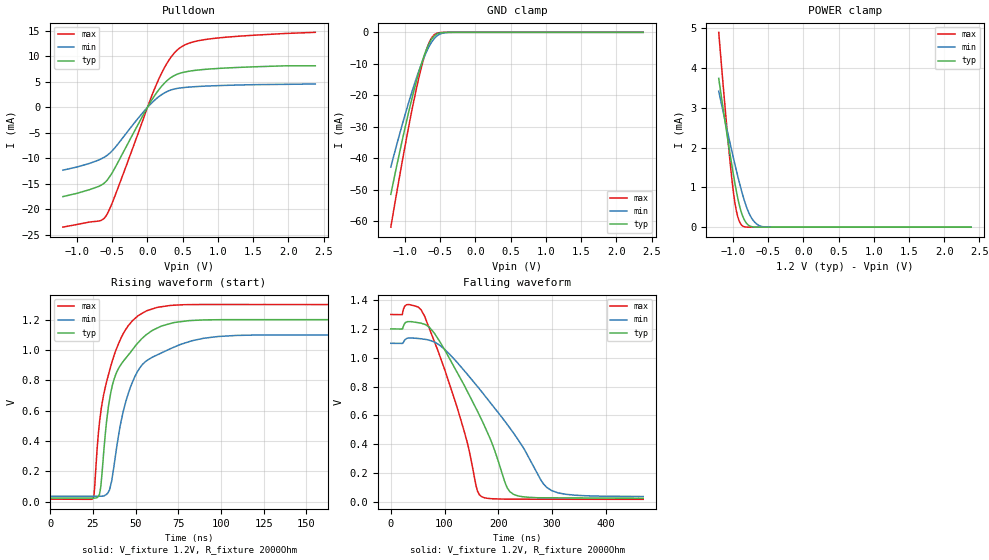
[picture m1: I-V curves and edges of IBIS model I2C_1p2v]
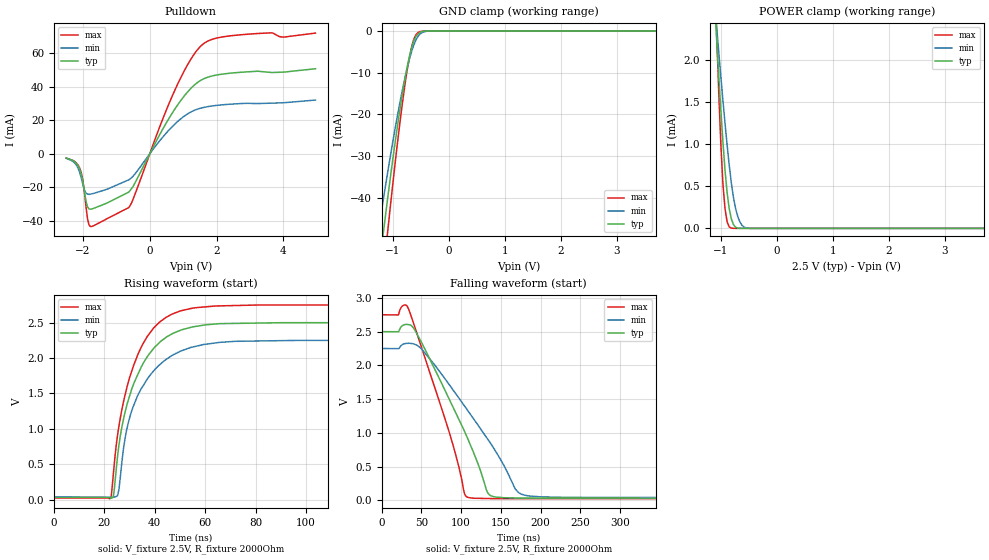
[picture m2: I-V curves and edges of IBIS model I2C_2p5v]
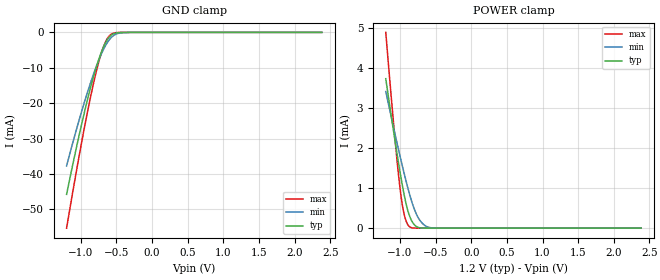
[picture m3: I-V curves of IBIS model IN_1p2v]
|Texas Instruments Incorporated
|Ultra Low Power Stereo Audio Codec with miniDSP, DirectPath Headphone,
| and Stereo Class-D Speaker Amplifier
|part#   Digital Voltage Range   Package-type   #pin
|TLV320AIC3212   1.1V to 3.6V   WCSP   81
[IBIS Ver]   4.0
[File name]   tlv320aic3212.ibs
[File Rev]   1.0
[Date]   09/07/2011
[Source]   Texas Instruments Incorporated.
   Analog-eLab, HPA
   12500 TI Blvd
   Dallas, TX -75243
   For Support e-mail: elab_ibis@list.ti.com
[Notes]   Revision History:
   1.0: 09/07/2011
- Initial version of the model
- Initial Model generated from simulations.
- Model not matched to measurements
- ccomp values are based on PVT conditions although listed in numerical order.
- Model names with a trailing _1p2v contains the model for 1.2V operaton.
- Model names with a trailing _1p8v contains the model for 1.8V operaton.
- Model names with a trailing _2p5v contains the model for 2.5V operaton.
- Model names with a trailing _3p3v contains the model for 3.3V operaton.
- Non monotinicity warnings related to combined Pullup/Pulldown of INOUT_xxxx and I2C_xxxx
  reflect the simulationresults.
[Disclaimer]
 This product is designed as an aid for customers of Texas Instruments.
 No warranties, either expressed or implied, with respect to this third
 party software (if any) or with respect to its fitness for any
 particular purpose is claimed by Texas Instruments or the author. The
 software (if any) is provided solely on an "as is" basis. The entire
 risk as to its quality and performance is with the customer
[Copyright] (C) Copyright 2012 Texas Instruments Incorporated.
   All rights reserved.
|   TLV320AIC3212
[Component]   tlv320aic3212
[Manufacturer] TI
[Package]   | 81 pin  package
| variable   typ   min   max
R_pkg   0.01   0.008   0.012
L_pkg   0.1nH   0.08nH   0.12nH
C_pkg   0.1pF   0.08pF   0.12pF
|-------------------------PIN------------------------------------------------
[Pin]   signal_name  model_name  R_pin  L_pin C_pin
A1   AVDD3_33   POWER   NA   NA   NA
A2   RECVSS   GND   NA   NA   NA
A3   RECVDD_33   POWER   NA   NA   NA
A4   HPR   TERM   NA   NA   NA
A5   VNEG   TERM   NA   NA   NA
A6   CPFCM   TERM   NA   NA   NA
A7   CPVDD_18   POWER   NA   NA   NA
A8   AVSS4   GND   NA   NA   NA
A9   SPKLP   TERM   NA   NA   NA
B1   MICDET   TERM   NA   NA   NA
B2   RECP   TERM   NA   NA   NA
B3   RECM   TERM   NA   NA   NA
B4   HVDD_18   POWER   NA   NA   NA
B5   HPL   TERM   NA   NA   NA
B6   CPVSS   GND   NA   NA   NA
B7   CPFCP   TERM   NA   NA   NA
B8   SLVDD   POWER   NA   NA   NA
B9   SLVSS   GND   NA   NA   NA
C1   IN4L   TERM   NA   NA   NA
C2   AVDD1_18   POWER   NA   NA   NA
C3   MICBIAS_EXT   TERM   NA   NA   NA
C4   MICBIAS   TERM   NA   NA   NA
C5   AVDD2_18   POWER   NA   NA   NA
C6   LOL   TERM   NA   NA   NA
C7   AVDD4_18   POWER   NA   NA   NA
C8   SPKLM   TERM   NA   NA   NA
C9   SPKRM   TERM   NA   NA   NA
D1   VREF_AUDIO   TERM   NA   NA   NA
D2   VREF_SAR   TERM   NA   NA   NA
D3   IN1L_AUX1   TERM   NA   NA   NA
D4   IN1R_AUX2   TERM   NA   NA   NA
D5   IN4R   TERM   NA   NA   NA
D6   HPVSS_SENSE   TERM   NA   NA   NA
D7   LOR   TERM   NA   NA   NA
D8   SRVSS   GND   NA   NA   NA
D9   SRVDD   POWER   NA   NA   NA
E1   IN3R   TERM   NA   NA   NA
E2   IN3L   TERM   NA   NA   NA
E3   AVSS   GND   NA   NA   NA
E4   AVSS1   GND   NA   NA   NA
E5   AVSS3   GND   NA   NA   NA
E6   AVSS2   GND   NA   NA   NA
E7   DVSS   GND   NA   NA   NA
E8   SPK_V   POWER   NA   NA   NA
E9   SPKRP   TERM   NA   NA   NA
F1   IN2L   TERM   NA   NA   NA
F2   IN2R   TERM   NA   NA   NA
F3   AVDD_18   POWER   NA   NA   NA
F4   DVSS   GND   NA   NA   NA
F5   GPI3   IN_PD   NA   NA   NA
F6   GPI2   IN   NA   NA   NA
F7   GPI4   IN_PD   NA   NA   NA
F8   IOVSS   GND   NA   NA   NA
F9   VBAT   TERM   NA   NA   NA
G1   MCLK1   IN   NA   NA   NA
G2   BCLK2   INOUT   NA   NA   NA
G3   DIN2   IN   NA   NA   NA
G4   WCLK2   INOUT   NA   NA   NA
G5   WCLK3   INOUT   NA   NA   NA
G6   DIN3   IN   NA   NA   NA
G7   SPI_SELECT  IN_PD   NA   NA   NA
G8   RESETB   IN   NA   NA   NA
G9   MCLK2   IN   NA   NA   NA
H1   BCLK1   INOUT   NA   NA   NA
H2   DOUT1   OUT_HOLD   NA   NA   NA
H3   IOVDD   POWER   NA   NA   NA
H4   SCL   I2C_IO   NA   NA   NA
H5   SDA   I2C_IO   NA   NA   NA
H6   GPO1   OUT   NA   NA   NA
H7   BCLK3   INOUT   NA   NA   NA
H8   GPIO2   INOUT   NA   NA   NA
H9   IOVDD   POWER   NA   NA   NA
J1   DIN1   IN   NA   NA   NA
J2   WCLK1   INOUT   NA   NA   NA
J3   DVDD   POWER   NA   NA   NA
J4   IOVSS   GND   NA   NA   NA
J5   GPI1   IN   NA   NA   NA
J6   DOUT2   OUT_HOLD   NA   NA   NA
J7   DOUT3   OUT_HOLD   NA   NA   NA
J8   GPIO1   INOUT   NA   NA   NA
J9   DVDD   POWER   NA   NA   NA
[Model Selector] I2C_IO
I2C_3p3v   I2C I/O with 3.3V operation.
I2C_2p5v   I2C I/O with 2.5V operation.
I2C_1p8v   I2C I/O with 1.8V operation.
I2C_1p2v   I2C I/O with 1.2V operation.
[Model Selector] IN
IN_3p3v   Input with 3.3V operation.
IN_2p5v   Input with 2.5V operation.
IN_1p8v   Input with 1.8V operation.
IN_1p2v   Input with 1.2V operation.
[Model Selector] IN_PD
IN_PD_3p3v  Input with 3.3V operation.
IN_PD_2p5v  Input with 2.5V operation.
IN_PD_1p8v  Input with 1.8V operation.
IN_PD_1p2v  Input with 1.2V operation.
[Model Selector] INOUT
INOUT_3p3v   I/O with 3.3V operation.
INOUT_2p5v   I/O with 2.5V operation.
INOUT_1p8v   I/O with 1.8V operation.
INOUT_1p2v   I/O with 1.2V operation.
[Model Selector] OUT
OUT_3p3v   Output with 3.3V operation.
OUT_2p5v   Output with 2.5V operation.
OUT_1p8v   Output with 1.8V operation.
OUT_1p2v   Output with 1.2V operation.
[Model Selector] OUT_HOLD
OUT_HOLD_3p3v   Output with 3.3V operation.
OUT_HOLD_2p5v   Output with 2.5V operation.
OUT_HOLD_1p8v   Output with 1.8V operation.
OUT_HOLD_1p2v   Output with 1.2V operation.
[Model Selector] TERM
TERM_3p3v   Termination with 3.3V operation.
TERM_2p5v   Termination with 2.5V operation.
TERM_1p8v   Termination with 1.8V operation.
TERM_1p2v   Termination with 1.2V operation.
|   TERM_1p2v
[Model]  TERM_1p2v
Model_type Terminator
C_comp   1fF   1fF   1fF
[Voltage Range]  1.2   1.1  1.3
[Temperature Range] 27   125   -40
|   TERM_1p8v
[Model]  TERM_1p8v
Model_type Terminator
C_comp   1fF   1fF   1fF
[Voltage Range]  1.8   1.65  1.95
[Temperature Range] 27   125   -40
|   TERM_2p5v
[Model]  TERM_2p5v
Model_type Terminator
C_comp   1fF   1fF   1fF
[Voltage Range]  2.5   2.25  2.75
[Temperature Range] 27   125   -40
|   TERM_3p3v
[Model]  TERM_3p3v
Model_type Terminator
C_comp   1fF   1fF   1fF
[Voltage Range]  3.3   2.7  3.6
[Temperature Range] 27   125   -40
| Models and submodels in the file (28): I2C_1p2v (I/O_open_drain), I2C_1p8v (I/O_open_drain), I2C_2p5v (I/O_open_drain), I2C_3p3v (I/O_open_drain), IN_1p2v (Input), IN_1p8v (Input), IN_2p5v (Input), IN_3p3v (Input), IN_PD_1p2v (Input), IN_PD_1p8v (Input), IN_PD_2p5v (Input), IN_PD_3p3v (Input), INOUT_1p2v (I/O), INOUT_1p8v (I/O), INOUT_2p5v (I/O), INOUT_3p3v (I/O), OUT_1p2v (Output), OUT_1p8v (Output), OUT_2p5v (Output), OUT_3p3v (Output), OUT_HOLD_1p2v (Output), OUT_HOLD_1p8v (Output), OUT_HOLD_2p5v (Output), OUT_HOLD_3p3v (Output), TERM_1p2v (Terminator), TERM_1p8v (Terminator), TERM_2p5v (Terminator), TERM_3p3v (Terminator)
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|   I2C_1p2v
[Model]   I2C_1p2v
Model_type   I/O_open_drain
Polarity   Non-Inverting
Enable   Active-High
Vinl = 0.12
Vinh = 1.08
Vmeas = 0.6
Vref = 0
Cref = 5pF
Rref = 2000
|   typ   min   max
C_comp   1.274pF   1.219pF   1.333pF
[Voltage Range]   1.2   1.1   1.3
[Temperature Range]   27   125   -40
[Pullup Reference]   1.2   1.1   1.3
[Pulldown Reference]   -0   -0   -0
[Power Clamp Reference]   1.2   1.1   1.3
[GND Clamp Reference]   -0   -0   -0
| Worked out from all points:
|   slope of the pulldown table from 0 to 0.18 V, typ, clamps not added: 47.5 ohm
|   GND clamp passes 1 mA (typ) near -0.58 V on its own axis
|   POWER clamp passes 1 mA (typ) near -0.96 V on its own axis
|   falling waveform, V_fixture 1.2V, R_fixture 2000Ohm: 20-80 % time 88.3ns typ, 123ns min, 62.1ns max; typ from 1.2 V to 0.024 V
|   rising waveform, V_fixture 1.2V, R_fixture 2000Ohm: 20-80 % time 14.7ns typ, 15.2ns min, 13.1ns max; typ from 0.024 V to 1.2 V
[Pulldown]
|   Voltage   I(typ)   I(min)   I(max)
-1.2V     -17.52mA   -12.33mA   -23.52mA
-660mV    -15.3mA    -10.14mA   -22.22mA
-588mV    -14.55mA   -9.571mA   -21.32mA
-534mV    -13.56mA   -8.98mA    -19.87mA
-444mV    -11.44mA   -7.63mA    -16.76mA
-84mV     -2.1mA     -1.335mA   -3.236mA
132mV     2.914mA    1.776mA    4.67mA
294mV     5.441mA    3.206mA    9.049mA
456mV     6.677mA    3.793mA    11.64mA
636mV     7.195mA    4.032mA    12.81mA
924mV     7.575mA    4.234mA    13.51mA
2.382V    8.16mA     4.595mA    14.74mA
[GND Clamp]
|   Voltage   I(typ)   I(min)   I(max)
-1.2V     -51.53mA   -42.82mA   -61.95mA
-1.11V    -41.81mA   -35.22mA   -50.18mA
-966mV    -27.21mA   -23.77mA   -32.33mA
-894mV    -20.51mA   -18.48mA   -24.05mA
-822mV    -14.35mA   -13.57mA   -16.43mA
-750mV    -8.941mA   -9.16mA    -9.735mA
-696mV    -5.556mA   -6.287mA   -5.617mA
-642mV    -2.944mA   -3.902mA   -2.598mA
-588mV    -1.249mA   -2.113mA   -881.8uA
-498mV    -172.7uA   -521.4uA   -72.82uA
-372mV    -4.652uA   -38.41uA   -629.2nA
2.382V    0A         0A         0A
[POWER Clamp]
|   Voltage   I(typ)   I(min)   I(max)
-1.2V     3.742mA    3.419mA    4.901mA
-1.074V   2.231mA    2.387mA    2.298mA
-1.002V   1.428mA    1.82mA     1.03mA
-966mV    1.06mA     1.547mA    562.3uA
-930mV    731.2uA    1.283mA    261.4uA
-894mV    461.7uA    1.032mA    95.6uA
-858mV    267uA      798.5uA    24.83uA
-804mV    94.07uA    498uA      2.256uA
-732mV    11.82uA    224.2uA    69.47nA
-660mV    942.6nA    77.54uA    0A
-570mV    25.2nA     10.87uA    0A
2.382V    0A         0A         0A
[Ramp]
R_load = 2000
|   typ   min   max
dV/dt_r   0.705406/1.46932e-008  0.638454/1.52438e-008  0.769932/1.30398e-008
dV/dt_f   0.705409/8.81291e-008   0.63829/1.23398e-007  0.769933/6.21317e-008
[Falling Waveform]
V_fixture = 1.2V
V_fixture_min = 1.1V
V_fixture_max = 1.3V
R_fixture = 2000Ohm
C_fixture = 0F
|   Time   V(typ)   V(min)   V(max)
0s        1.2V       1.1V       1.3V
32.69ns   1.251V     1.136V     1.369V
62.72ns   1.232V     1.128V     1.29V
120.1ns   920.9mV    981.3mV    694.6mV
161.3ns   629.2mV    800.4mV    74.84mV
169.6ns   565.2mV    761.9mV    34.22mV
216.7ns   96.76mV    537mV      17.74mV
228.5ns   51.31mV    476.9mV    17.7mV
299.2ns   27.33mV    77.85mV    17.43mV
470ns     24.32mV    36.18mV    16.78mV
[Rising Waveform]
V_fixture = 1.2V
V_fixture_min = 1.1V
V_fixture_max = 1.3V
R_fixture = 2000Ohm
C_fixture = 0F
|   Time   V(typ)   V(min)   V(max)
0s        24.32mV    35.9mV     16.78mV
24.99ns   24.02mV    35.98mV    20.42mV
29.9ns    136.2mV    36mV       617.3mV
34.13ns   633.5mV    65.85mV    839.6mV
37.53ns   812.9mV    252.1mV    970.6mV
42.58ns   923.8mV    589mV      1.105V
48.06ns   1.001V     786.7mV    1.193V
62.72ns   1.146V     968.9mV    1.282V
109.1ns   1.201V     1.097V     1.301V
470ns     1.2V       1.1V       1.3V
|   I2C_2p5v
[Model]   I2C_2p5v
Model_type   I/O_open_drain
Polarity   Non-Inverting
Enable   Active-High
Vinl = 0.75
Vinh = 1.75
Vmeas = 1.25
Vref = 0
Cref = 5pF
Rref = 2000
|   typ   min   max
C_comp   1.274pF   1.219pF   1.333pF
[Voltage Range]   2.5   2.25   2.75
[Temperature Range]   27   125   -40
[Pullup Reference]   2.5   2.25   2.75
[Pulldown Reference]   -0   -0   -0
[Power Clamp Reference]   2.5   2.25   2.75
[GND Clamp Reference]   -0   -0   -0
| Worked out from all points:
|   slope of the pulldown table from 0 to 0.375 V, typ, clamps not added: 26.4 ohm
|   GND clamp passes 1 mA (typ) near -0.57 V on its own axis
|   POWER clamp passes 1 mA (typ) near -0.96 V on its own axis
|   falling waveform, V_fixture 2.5V, R_fixture 2000Ohm: 20-80 % time 57.5ns typ, 76.1ns min, 43.6ns max; typ from 2.5 V to 0.031 V
|   rising waveform, V_fixture 2.5V, R_fixture 2000Ohm: 20-80 % time 11.8ns typ, 12.5ns min, 11.3ns max; typ from 0.031 V to 2.5 V
[Pulldown]
|   Voltage   I(typ)   I(min)   I(max)
-2.5V     -2.526mA   -2.66mA    -2.537mA
-2.237V   -4.926mA   -5.666mA   -4.77mA
-2.087V   -9.625mA   -11.74mA   -9.035mA
-2.013V   -15.52mA   -17.53mA   -14.79mA
-1.9V     -28.98mA   -23.51mA   -33.15mA
-1.825V   -32.66mA   -24.09mA   -41.94mA
-1.675V   -32.39mA   -23.49mA   -42.71mA
-625mV    -22.72mA   -15.42mA   -31.93mA
725mV     25.83mA    17.19mA    36.69mA
1.55V     43.97mA    27.3mA     64.52mA
2.525V    48.19mA    29.68mA    70.44mA
4.963V    50.63mA    32mA       71.83mA
[GND Clamp]
|   Voltage   I(typ)   I(min)   I(max)
-2.5V     -395.5mA   -330.9mA   -444.7mA
-1.375V   -71.35mA   -58.36mA   -85.71mA
-1.188V   -50.16mA   -41.75mA   -60.29mA
-1.15V    -46.08mA   -38.56mA   -55.36mA
-1.113V   -42.07mA   -35.43mA   -50.5mA
-1.075V   -38.14mA   -32.35mA   -45.71mA
-887.5mV  -19.93mA   -18.02mA   -23.34mA
-737.5mV  -8.099mA   -8.458mA   -8.701mA
-625mV    -2.309mA   -3.27mA    -1.918mA
-550mV    -742.7uA   -1.242mA   -338.4uA
-287.5mV  -254.6nA   -5.008uA   -31.57nA
4.963V    0A         0A         0A
[POWER Clamp]
|   Voltage   I(typ)   I(min)   I(max)
-2.5V     20.66mA    14.8mA     34.71mA
-1.113V   2.682mA    2.698mA    3.063mA
-1.075V   2.242mA    2.395mA    2.317mA
-1V       1.406mA    1.805mA    1mA
-962.5mV  1.026mA    1.521mA    525.7uA
-925mV    689.7uA    1.247mA    231.4uA
-887.5mV  420.9uA    988.2uA    76.84uA
-812.5mV  113.7uA    540.4uA    3.319uA
-700mV    3.918uA    146.5uA    40.28nA
-625mV    247.3nA    39.26uA    0A
-512.5mV  0A         2.416uA    0A
4.963V    0A         0A         0A
[Ramp]
R_load = 2000
|   typ   min   max
dV/dt_r   1.48138/1.18177e-008   1.32568/1.24678e-008   1.63535/1.12722e-008
dV/dt_f   1.48139/5.7451e-008   1.32569/7.60824e-008   1.63535/4.35846e-008
[Falling Waveform]
V_fixture = 2.5V
V_fixture_min = 2.25V
V_fixture_max = 2.75V
R_fixture = 2000Ohm
C_fixture = 0F
|   Time   V(typ)   V(min)   V(max)
0s        2.5V       2.25V      2.75V
33.44ns   2.604V     2.327V     2.844V
50.29ns   2.335V     2.241V     2.258V
85.86ns   1.476V     1.7V       973.4mV
104.3ns   1.019V     1.396V     94.24mV
107.1ns   945.1mV    1.35V      51.42mV
133.6ns   106.2mV    901.3mV    26.95mV
168ns     35.18mV    167.6mV    25.37mV
176.8ns   33.5mV     86.17mV    25.34mV
470ns     31.02mV    40.52mV    24.42mV
[Rising Waveform]
V_fixture = 2.5V
V_fixture_min = 2.25V
V_fixture_max = 2.75V
R_fixture = 2000Ohm
C_fixture = 0F
|   Time   V(typ)   V(min)   V(max)
0s        31.02mV    40.52mV    24.42mV
22.61ns   24.73mV    36.32mV    22.9mV
23.85ns   103.7mV    36.09mV    457.1mV
25.36ns   639.4mV    67.87mV    931.3mV
26.72ns   976.1mV    445.2mV    1.224V
29.13ns   1.358V     1.027V     1.608V
33.44ns   1.779V     1.484V     2.061V
41.98ns   2.223V     1.906V     2.509V
54.82ns   2.439V     2.154V     2.703V
470ns     2.5V       2.25V      2.75V
|   IN_1p2v
[Model]   IN_1p2v
Model_type   Input
Vinl = 1.08
Vinh = 0.12
|   typ   min   max
C_comp   1.095pF   1.082pF   1.133pF
[Voltage Range]   1.2   1.1   1.3
[Temperature Range]   27   125   -40
[Power Clamp Reference]   1.2   1.1   1.3
[GND Clamp Reference]   -0   -0   -0
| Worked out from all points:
|   GND clamp passes 1 mA (typ) near -0.58 V on its own axis
|   POWER clamp passes 1 mA (typ) near -0.96 V on its own axis
[GND Clamp]
|   Voltage   I(typ)   I(min)   I(max)
-1.2V     -45.78mA   -37.73mA   -55.33mA
-1.11V    -37.06mA   -30.96mA   -44.72mA
-984mV    -25.55mA   -22.02mA   -30.58mA
-894mV    -18.01mA   -16.12mA   -21.24mA
-822mV    -12.53mA   -11.79mA   -14.42mA
-750mV    -7.751mA   -7.917mA   -8.472mA
-696mV    -4.78mA    -5.405mA   -4.842mA
-642mV    -2.508mA   -3.332mA   -2.212mA
-588mV    -1.053mA   -1.79mA    -741uA
-480mV    -90.52uA   -311.7uA   -33.57uA
-300mV    -348.8nA   -5.721uA   -17.65nA
2.382V    0A         0A         0A
[POWER Clamp]
|   Voltage   I(typ)   I(min)   I(max)
-1.2V     3.742mA    3.419mA    4.901mA
-1.074V   2.231mA    2.387mA    2.298mA
-1.002V   1.428mA    1.82mA     1.03mA
-966mV    1.06mA     1.547mA    562.3uA
-930mV    731.2uA    1.283mA    261.4uA
-894mV    461.8uA    1.032mA    95.61uA
-858mV    267uA      798.5uA    24.84uA
-804mV    94.08uA    498uA      2.263uA
-732mV    11.82uA    224.2uA    76.87nA
-660mV    950.1nA    77.55uA    837.8pA
-570mV    32.74nA    10.88uA    0A
2.382V    0A         0A         0A
